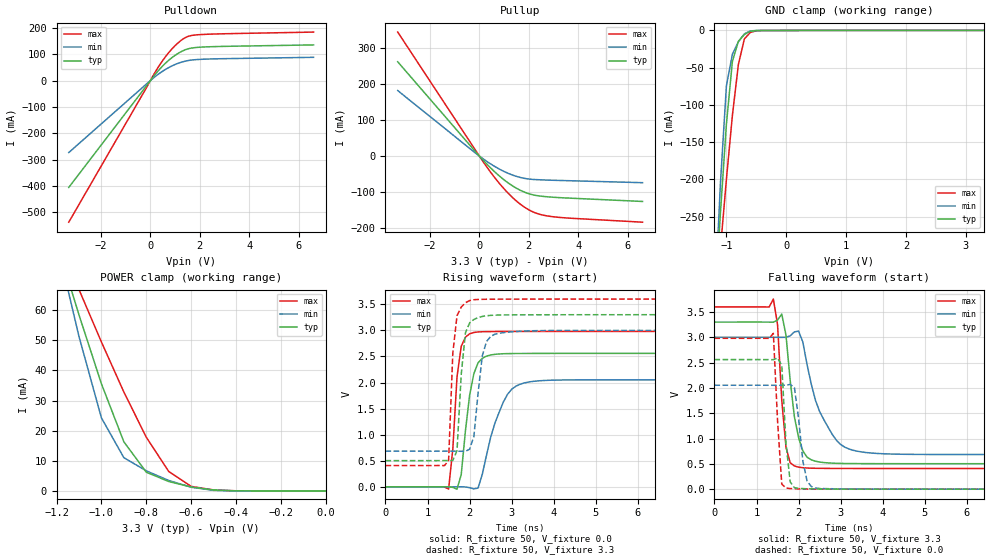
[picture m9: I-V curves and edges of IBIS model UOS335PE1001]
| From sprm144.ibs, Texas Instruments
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[Model]   UOS335PE1001
| 3_state with a pulldn
Model_type   3-state
Enable   Active-Low
Polarity   Non-Inverting
| signals   A, GZ, Y
Vmeas = 1.5
|   typ   min   max
C_comp   2.373p   2.375p   2.367p
|   typ   min   max
[Temperature Range]   25   -40   125
|   typ   min   max
[Voltage Range]   3.30V   3.00V   3.60V
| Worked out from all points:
|   slope of the pulldown table from 0 to 0.495 V, typ, clamps not added: 8.97 ohm
|   slope of the pullup table from 0 to 0.495 V, typ, clamps not added: 13.9 ohm
|   GND clamp passes 1 mA (typ) near -0.59 V on its own axis
|   POWER clamp passes 1 mA (typ) near -0.57 V on its own axis
|   rising waveform, R_fixture 50, V_fixture 0.0: 20-80 % time 237ps typ, 464ps min, 164ps max; typ from 0 V to 2.56 V
|   falling waveform, R_fixture 50, V_fixture 3.3: 20-80 % time 255ps typ, 570ps min, 157ps max; typ from 3.3 V to 0.503 V
|   rising waveform, R_fixture 50, V_fixture 3.3: 20-80 % time 148ps typ, 188ps min, 129ps max; typ from 0.503 V to 3.3 V
|   falling waveform, R_fixture 50, V_fixture 0.0: 20-80 % time 126ps typ, 178ps min, 120ps max; typ from 2.56 V to 0 V
[Pulldown]
|   Voltage   I(typ)   I(min)   I(max)
-3.3V     -405.5mA   -273.2mA   -537.5mA
300mV     35.25mA    22.75mA    48.21mA
600mV     64.95mA    41.72mA    89.2mA
800mV     81.64mA    52.25mA    112.5mA
1.2V      107.5mA    68.13mA    149.4mA
1.5V      119.8mA    75.48mA    166.9mA
2V        126.6mA    80.41mA    174.4mA
6.6V      135.3mA    88.27mA    184mA
[GND_clamp]
|   Voltage   I(typ)   I(min)   I(max)
-3.3V     -3.476A    -4.508A    -2.62A
-1.2V     -377.4mA   -375.8mA   -391.1mA
-1.1V     -245.2mA   -205.2mA   -293.5mA
-1V       -125.7mA   -74.36mA   -199.9mA
-900mV    -41.55mA   -31.84mA   -114.1mA
-800mV    -14.66mA   -15.3mA    -45.7mA
-700mV    -5.342mA   -4.518mA   -11.36mA
-600mV    -1.076mA   -585uA     -2.664mA
-500mV    -138.6uA   -92.96uA   -491uA
-400mV    -41.17uA   -55.74uA   -77.59uA
3.3V      100.3uA    176.6uA    56.17uA
[Pullup]
|   Voltage   I(typ)   I(min)   I(max)
-3.3V     261.2mA    181.5mA    343.6mA
-200mV    15.59mA    10.64mA    20.79mA
300mV     -22.18mA   -14.8mA    -30.05mA
700mV     -48.7mA    -32mA      -66.54mA
1V        -66mA      -42.81mA   -90.87mA
1.3V      -80.83mA   -51.65mA   -112.3mA
1.6V      -92.95mA   -58.38mA   -130.4mA
1.9V      -102.1mA   -62.82mA   -145.1mA
2.2V      -108.1mA   -65mA      -155.8mA
2.8V      -113.3mA   -66.81mA   -166.6mA
3.6V      -116.6mA   -68.38mA   -172mA
6.6V      -125.9mA   -73.9mA    -183.4mA
[POWER_clamp]
|   Voltage   I(typ)   I(min)   I(max)
-3.3V     636.9mA    822.3mA    484mA
-1.2V     82.8mA     82.87mA    84.8mA
-1.1V     58.47mA    51.3mA     66.89mA
-1V       35.58mA    24.26mA    49.46mA
-900mV    16.31mA    11.04mA    32.84mA
-800mV    6.225mA    6.672mA    17.82mA
-700mV    3.121mA    3.469mA    6.452mA
-600mV    1.315mA    1.222mA    1.513mA
-500mV    313uA      181.3uA    320.7uA
-400mV    30.66uA    9.589uA    44.96uA
0V        799.4pA    133.2pA    19.14nA
[Ramp]
|   I(typ)   I(min)   I(max)
dV/dt_r   1.536/0.229n   1.231/0.462n   1.788/0.142n
dV/dt_f   1.678/0.253n   1.390/0.569n   1.915/0.148n
[Rising Waveform]
R_fixture = 50
V_fixture = 0.0
|  pu_on
|  TIME   V(typ)   V(min)   V(max)
0s        1nV        12nV       1nV
1.5ns     2.163mV    339uV      -41.63mV
1.6ns     -9.657mV   651.8uV    723.8mV
1.7ns     -44.31mV   1.106mV    2.11V
1.8ns     235.7mV    1.688mV    2.695V
2ns       1.76V      -15.57mV   2.935V
2.3ns     2.464V     239.1mV    2.974V
2.8ns     2.552V     1.625V     2.978V
3.2ns     2.557V     1.967V     2.979V
10ns      2.559V     2.052V     2.98V
[Falling Waveform]
R_fixture = 50
V_fixture = 3.3
V_fixture_min = 3.0
V_fixture_max = 3.6
|  pd_on
|  TIME   V(typ)   V(min)   V(max)
0s        3.3V       3V         3.6V
1.4ns     3.297V     3V         3.755V
1.5ns     3.34V      2.999V     3.248V
1.6ns     3.46V      2.998V     1.756V
1.7ns     3.044V     2.999V     828.2mV
1.9ns     1.429V     3.107V     458mV
2.2ns     633mV      2.466V     417.7mV
2.5ns     535.8mV    1.532V     411.4mV
3.2ns     506.2mV    793.1mV    408.8mV
10ns      502.8mV    683.6mV    408.3mV
[Rising Waveform]
R_fixture = 50
V_fixture = 3.3
V_fixture_min = 3.0
V_fixture_max = 3.6
|  pd_off
|  TIME   V(typ)   V(min)   V(max)
0s        502.8mV    683.6mV    408.3mV
1.5ns     503.4mV    684.3mV    506.7mV
1.6ns     504.8mV    684.2mV    2.565V
1.7ns     695.4mV    683.7mV    3.281V
1.8ns     2.152V     681.8mV    3.447V
2ns       3.144V     721.2mV    3.571V
2.1ns     3.208V     964.3mV    3.587V
2.3ns     3.267V     2.51V      3.595V
2.6ns     3.292V     2.927V     3.597V
10ns      3.3V       3V         3.6V
[Falling Waveform]
R_fixture = 50
V_fixture = 0.0
|  pu_off
|  TIME   V(typ)   V(min)   V(max)
0s        2.559V     2.053V     2.98V
1.4ns     2.557V     2.052V     3.078V
1.5ns     2.59V      2.051V     1.346V
1.6ns     2.446V     2.051V     99.56mV
1.7ns     910.5mV    2.054V     22.86mV
1.8ns     143.4mV    2.069V     12.12mV
1.9ns     30.18mV    2.008V     7.773mV
2.2ns     8.053mV    165.6mV    2.623mV
2.4ns     4.568mV    23.16mV    1.516mV
10ns      45nV       4.306uV    1.216uV
